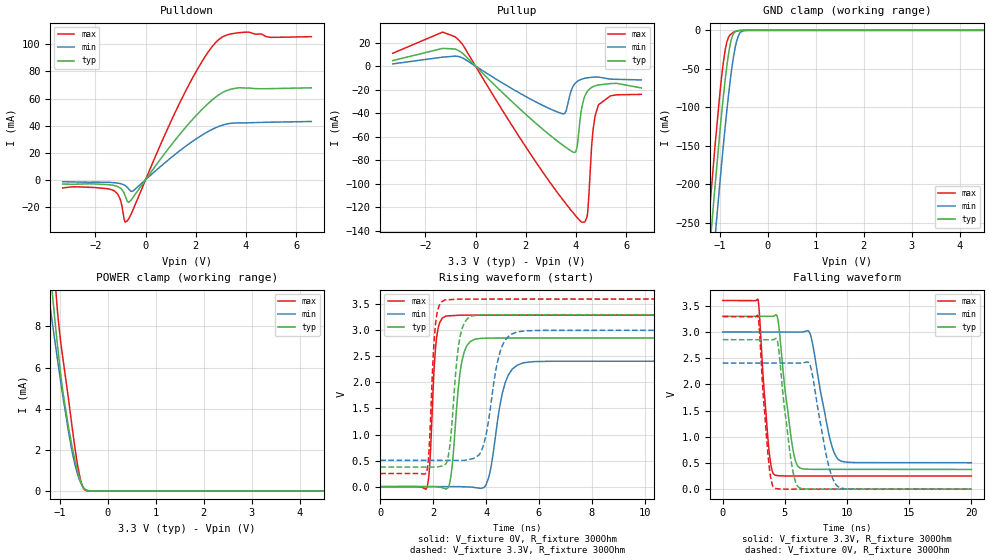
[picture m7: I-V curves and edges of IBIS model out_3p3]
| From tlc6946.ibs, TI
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|   out_3p3 Model
[Model]   out_3p3
Model_type   3-state
Polarity   Non-Inverting
Vmeas = 1.65
Vref = 0
Cref = 2pF
Rref = 100000
|   typ   min   max
C_comp   3.799pF   3.595pF   3.887pF
|  Where Nom  PVT is Nominal Process, 3.3V,   27C
|   Fast PVT is Strong Process,  3.6V,   -40C
|   Slow PVT is Weak Process,   3.0V,   105C
[Voltage Range]   3.3   3   3.6
|Junction Temperature
[Temperature Range]   27   105   -40
[Pullup Reference]   3.3   3   3.6
[Pulldown Reference]   0   0   -0
[Power Clamp Reference]   3.3   3   3.6
[GND Clamp Reference]   0   0   0
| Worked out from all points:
|   slope of the pulldown table from 0 to 0.495 V, typ, clamps not added: 38.9 ohm
|   slope of the pullup table from 0 to 0.495 V, typ, clamps not added: 47.1 ohm
|   GND clamp passes 1 mA (typ) near -0.65 V on its own axis
|   POWER clamp passes 1 mA (typ) near -0.64 V on its own axis
|   falling waveform, V_fixture 3.3V, R_fixture 300Ohm: 20-80 % time 834ps typ, 1.15ns min, 595ps max; typ from 3.3 V to 0.377 V
|   rising waveform, V_fixture 0V, R_fixture 300Ohm: 20-80 % time 294ps typ, 465ps min, 190ps max; typ from 0 V to 2.85 V
|   rising waveform, V_fixture 3.3V, R_fixture 300Ohm: 20-80 % time 297ps typ, 486ps min, 187ps max; typ from 0.377 V to 3.3 V
|   falling waveform, V_fixture 0V, R_fixture 300Ohm: 20-80 % time 818ps typ, 1.09ns min, 589ps max; typ from 2.85 V to 0 V
[Pulldown]
|   Voltage   I(typ)   I(min)   I(max)
-3.3V     -3.201mA   -1.471mA   -6.042mA
-1.261V   -4.226mA   -2.173mA   -8.089mA
-1.023V   -5.947mA   -2.782mA   -13.74mA
-815.1mV  -11.74mA   -4.27mA    -31.36mA
-726mV    -16.08mA   -5.706mA   -30.32mA
-597.3mV  -15.44mA   -8.32mA    -26.21mA
1.541V    37.51mA    23.94mA    63.51mA
2.788V    60.97mA    38.4mA     101.3mA
3.204V    65.67mA    41.04mA    106.7mA
4.036V    67.7mA     42.03mA    109mA
4.986V    67.29mA    42.49mA    105.1mA
6.6V      67.91mA    43.04mA    105.7mA
[GND Clamp]
|   Voltage   I(typ)   I(min)   I(max)
-3.3V     -1.946A    -1.939A    -1.96A
-1.251V   -314mA     -379.5mA   -262.6mA
-1.211V   -283.8mA   -349.9mA   -232mA
-1.122V   -217.5mA   -284.3mA   -165.1mA
-1.102V   -203.1mA   -269.9mA   -150.8mA
-983.4mV  -121mA     -186.5mA   -71.8mA
-894.3mV  -66.79mA   -128.2mA   -27.37mA
-785.4mV  -18.6mA    -65.74mA   -5.899mA
-676.5mV  -1.703mA   -21.01mA   -1.454mA
-587.4mV  -193.7uA   -3.997mA   -229.8uA
-448.8mV  -4.904uA   -96.06uA   -3.991uA
6.6V      0A         0A         0A
[Pullup]
|   Voltage   I(typ)   I(min)   I(max)
-3.3V     4.753mA    1.94mA     10.98mA
-1.31V    15.14mA    7.703mA    29.01mA
-676.5mV  13.24mA    8.231mA    22.4mA
3.472V    -67.16mA   -40.52mA   -113.6mA
3.897V    -73.27mA   -16.61mA   -125mA
4.036V    -69.42mA   -13.22mA   -128.5mA
4.234V    -34.72mA   -10.98mA   -132.7mA
4.442V    -21.72mA   -9.935mA   -127.9mA
4.67V     -17.5mA    -9.371mA   -55.93mA
4.887V    -16.01mA   -9.246mA   -33.28mA
5.362V    -14.82mA   -10.99mA   -25.33mA
6.6V      -18.48mA   -11.71mA   -23.98mA
[POWER Clamp]
|   Voltage   I(typ)   I(min)   I(max)
-3.3V     68.67mA    47.35mA    109.4mA
-1.3V     13.21mA    10.64mA    17.99mA
-1.191V   10.45mA    8.763mA    13.57mA
-1.162V   9.713mA    8.258mA    12.44mA
-1.092V   8.057mA    7.096mA    10.01mA
-1.063V   7.376mA    6.605mA    9.105mA
-943.8mV  4.945mA    4.701mA    6.559mA
-815.1mV  3.029mA    2.815mA    4.388mA
-607.2mV  749.7uA    646.8uA    955uA
-537.9mV  277.9uA    270.7uA    282.6uA
-458.7mV  39.85uA    58.11uA    21.81uA
6.6V      0A         0A         0A
[Ramp]
R_load = 300
|   typ   min   max
dV/dt_r   1.71176/2.93993e-10   1.44432/4.61066e-10   1.97509/1.89848e-10
dV/dt_f   1.75398/8.34501e-10   1.49712/1.1537e-09   2.00907/5.9473e-10
[Falling Waveform]
V_fixture = 3.3V
V_fixture_min = 3V
V_fixture_max = 3.6V
R_fixture = 300Ohm
C_fixture = 0F
|   Time   V(typ)   V(min)   V(max)
0s        3.3V       3V         3.6V
2.837ns   3.299V     2.999V     3.62V
3.688ns   3.298V     2.999V     830mV
4.166ns   3.309V     2.999V     275.4mV
4.457ns   3.209V     2.999V     257.5mV
5.586ns   846.4mV    2.999V     251.9mV
6.183ns   407.9mV    2.999V     251.9mV
7.049ns   379.3mV    2.955V     251.9mV
9.298ns   377.3mV    569.3mV    251.8mV
20ns      376.7mV    504.8mV    251.6mV
[Rising Waveform]
V_fixture = 0V
V_fixture_min = 0V
V_fixture_max = 0V
R_fixture = 300Ohm
C_fixture = 0F
|   Time   V(typ)   V(min)   V(max)
0s        -48nV      -48.63nV   -451.3nV
1.771ns   124.4uV    242.5uV    -9.861mV
2.114ns   -4.59mV    289.4uV    2.786V
2.471ns   -41.71mV   338.3uV    3.274V
2.673ns   206.9mV    365.9uV    3.28V
3.086ns   2.405V     -1.593mV   3.292V
3.577ns   2.829V     -16.99mV   3.292V
4.742ns   2.853V     2.02V      3.292V
5.404ns   2.853V     2.375V     3.292V
20ns      2.853V     2.407V     3.292V
[Rising Waveform]
V_fixture = 3.3V
V_fixture_min = 3V
V_fixture_max = 3.6V
R_fixture = 300Ohm
C_fixture = 0F
|   Time   V(typ)   V(min)   V(max)
0s        376.7mV    504.8mV    251.6mV
1.74ns    375mV      504.2mV    266.3mV
2.089ns   374.6mV    504mV      3.115V
2.434ns   419.7mV    503.9mV    3.582V
3.004ns   2.841V     503.7mV    3.6V
3.481ns   3.276V     534.1mV    3.6V
3.953ns   3.297V     892.1mV    3.6V
4.573ns   3.3V       2.65V      3.6V
5.17ns    3.3V       2.968V     3.6V
20ns      3.3V       3V         3.6V
[Falling Waveform]
|Gnd
V_fixture = 0V
V_fixture_min = 0V
V_fixture_max = 0V
R_fixture = 300Ohm
C_fixture = 0F
|   Time   V(typ)   V(min)   V(max)
0s        2.853V     2.407V     3.292V
2.837ns   2.852V     2.407V     3.311V
3.637ns   2.852V     2.407V     672.7mV
4.131ns   2.857V     2.406V     27.23mV
4.457ns   2.756V     2.406V     4.811mV
5.586ns   420.1mV    2.406V     343.8uV
6.14ns    31.86mV    2.406V     330.6uV
7.049ns   2.198mV    2.352V     308.9uV
9.202ns   616.1uV    62.93mV    257.5uV
20ns      -136.9nV   -48.64nV   -424.7nV
